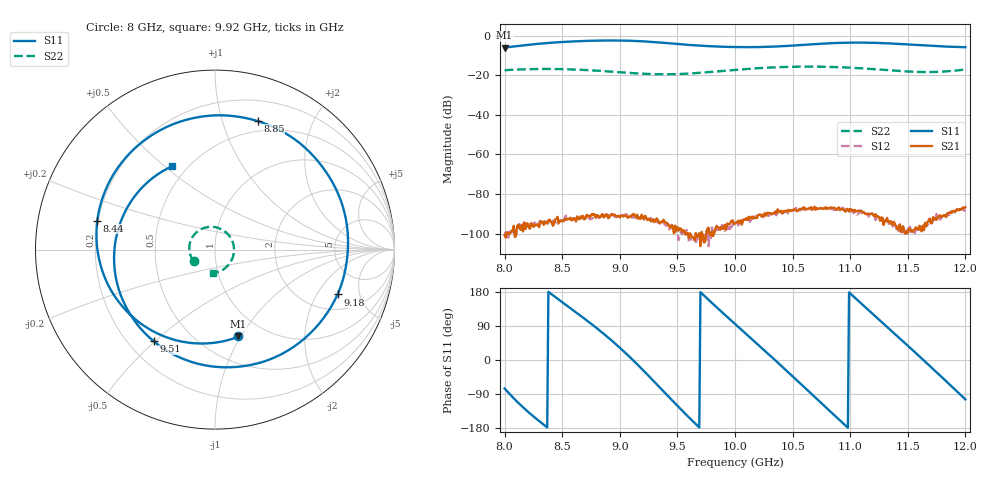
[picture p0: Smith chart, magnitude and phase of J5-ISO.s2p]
!Keysight Technologies,N5234A,MY52241180,A.10.60.03
!Date: Tuesday, May 30, 2023 15:21:41
!Correction: S11(Full 2 Port(1,2))
!S21(Full 2 Port(1,2))
!S12(Full 2 Port(1,2))
!S22(Full 2 Port(1,2))
!S2P File: Measurements: S11, S21, S12, S22:
# Hz S  dB  R 50
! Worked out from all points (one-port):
!   401 points, 8 GHz to 12 GHz, reference 50 ohm
!   lowest |S11| = -6.0 dB at 8 GHz (marker M1), VSWR 3.00, Z = 37.6 - j48.6 ohm
!   |S11| at or under -10 dB: nowhere
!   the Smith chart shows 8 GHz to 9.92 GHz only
!   S11 on the Smith chart (normalised r, x): 8 GHz: 0.75, -0.97; 8.44 GHz: 0.20, +0.12; 8.85 GHz: 0.39, +1.31; 9.18 GHz: 2.89, -3.06; 9.51 GHz: 0.30, -0.50; 9.92 GHz: 0.42, +0.53
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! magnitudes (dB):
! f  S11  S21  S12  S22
! 8 GHz  -6.0  -100.7  -101.1  -17.5
! 8.21 GHz  -4.6  -96.9  -96.5  -16.9
! 8.44 GHz  -3.4  -92.8  -92.9  -16.8
! 8.67 GHz  -2.7  -91.9  -92.4  -17.2
! 8.85 GHz  -2.4  -90.1  -91.6  -17.8
! 9.03 GHz  -2.5  -91.2  -91.4  -18.6
! 9.18 GHz  -2.8  -92.5  -91.9  -19.1
! 9.34 GHz  -3.4  -94.4  -94.5  -19.5
! 9.51 GHz  -4.2  -98.5  -103.3  -19.4
! 9.73 GHz  -5.2  -104.4  -104.0  -18.6
! 9.92 GHz  -5.6  -97.9  -98.2  -17.6
! 10 GHz  -5.7  -95.0  -94.5  -17.3
! 10.31 GHz  -5.6  -89.8  -89.8  -16.1
! 10.67 GHz  -4.3  -87.9  -87.9  -15.6
! 10.85 GHz  -3.7  -87.1  -87.2  -15.8
! 11 GHz  -3.5  -87.5  -88.8  -16.2
! 11.18 GHz  -3.6  -90.1  -91.1  -16.8
! 11.34 GHz  -3.9  -94.2  -95.7  -17.5
! 11.54 GHz  -4.6  -99.1  -99.2  -18.2
! 11.69 GHz  -5.1  -92.4  -93.7  -18.4
! 11.83 GHz  -5.5  -91.6  -90.8  -18.0
! 12 GHz  -5.8  -86.8  -88.0  -17.1
